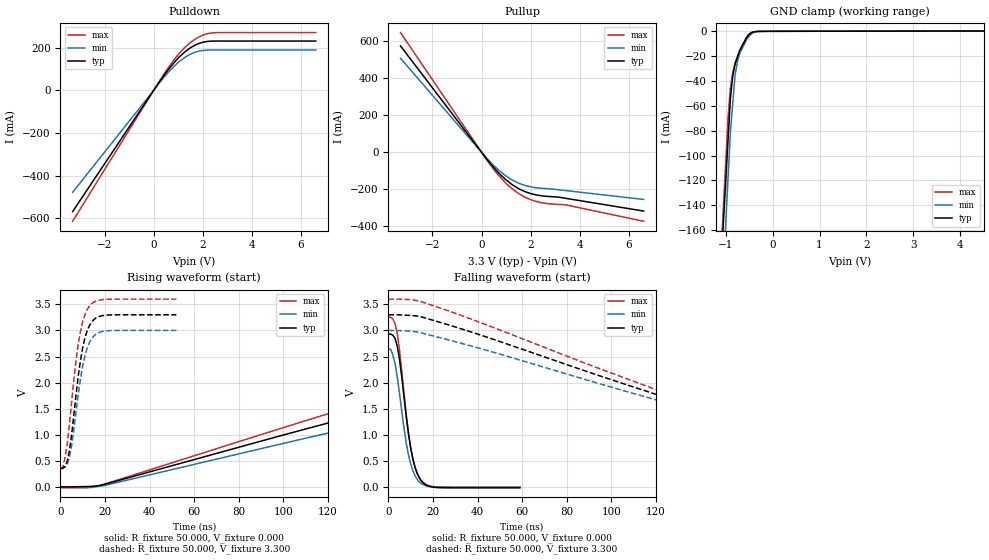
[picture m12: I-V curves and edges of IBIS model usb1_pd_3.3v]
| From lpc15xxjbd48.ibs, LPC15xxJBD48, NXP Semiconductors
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[Model]   usb1_pd_3.3v
Model_type I/O
Vinl=9.900E-01
Vinh=2.310E+00
Vref=0.000E+00
Rref=1.000E+06
Cref=0.000E+00
Vmeas=1.650E+00
C_comp   2.000E-12   2.000E-12   2.000E-12
[Voltage Range]   3.300E+00   3.000E+00   3.600E+00
[POWER Clamp Reference]   3.300E+00   3.000E+00   3.600E+00
[GND Clamp Reference]   0.000E+00   0.000E+00   0.000E+00
[Pullup Reference]   3.300E+00   3.000E+00   3.600E+00
[Pulldown Reference]   0.000E+00   0.000E+00   0.000E+00
[Temperature Range]   25   85   -40
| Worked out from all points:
|   slope of the pulldown table from 0 to 0.495 V, typ, clamps not added: 6.06 ohm
|   slope of the pullup table from 0 to 0.495 V, typ, clamps not added: 6.04 ohm
|   GND clamp passes 1 mA (typ) near -0.44 V on its own axis
|   rising waveform, R_fixture 50.000, V_fixture 0.000: 20-80 % time 164ns typ, 173ns min, 155ns max; typ from 0 V to 2.95 V
|   falling waveform, R_fixture 50.000, V_fixture 0.000: 20-80 % time 5.51ns typ, 5.54ns min, 5.45ns max; typ from 2.93 V to -0.014 V
|   rising waveform, R_fixture 50.000, V_fixture 3.300: 20-80 % time 5.37ns typ, 5.43ns min, 5.35ns max; typ from 0.352 V to 3.3 V
|   falling waveform, R_fixture 50.000, V_fixture 3.300: 20-80 % time 127ns typ, 132ns min, 123ns max; typ from 3.3 V to 0.352 V
[GND Clamp]
-3.3V     -1.665A    -1.867A    -1.78A
-950mV    -88mA      -118.7mA   -70.2mA
-900mV    -54.45mA   -81.5mA    -45.76mA
-850mV    -36.23mA   -58.43mA   -32.88mA
-800mV    -26.46mA   -35.35mA   -25.59mA
-750mV    -21mA      -24.36mA   -20.37mA
-700mV    -15.55mA   -17.9mA    -15.15mA
-550mV    -4.778mA   -6.346mA   -4.234mA
-450mV    -1.105mA   -1.932mA   -913.8uA
-350mV    -204.8uA   -365.7uA   -198.6uA
-150mV    -14.97uA   -25.94uA   -16.54uA
6.6V      390.1uA    400uA      390.5uA
[Power Clamp]
-3.3V     0A         0A         0A
0V        0A         0A         0A
3.3V      0A         0A         0A
6.6V      0A         0A         0A
[Pullup]
-3.3V     573.9mA    507.4mA    646.2mA
260mV     -45.14mA   -39.12mA   -50.35mA
720mV     -114.4mA   -98.69mA   -128mA
1.02V     -151.1mA   -130mA     -170.2mA
1.28V     -177.4mA   -151.7mA   -200.2mA
1.8V      -213.8mA   -180.2mA   -244.2mA
2.34V     -232.8mA   -193.1mA   -269.2mA
2.74V     -238.6mA   -196.9mA   -277.9mA
3.44V     -248.8mA   -206.9mA   -284.2mA
6.6V      -317.3mA   -254.6mA   -372.5mA
[Pulldown]
-3.3V     -569.7mA   -479mA     -615.1mA
420mV     69.92mA    61.22mA    76.39mA
1V        151.6mA    131.1mA    167.7mA
1.48V     198.8mA    169.2mA    223.1mA
1.94V     224mA      186.5mA    256.1mA
2.44V     231.7mA    189.6mA    270.6mA
6.6V      231.7mA    189.6mA    271.6mA
[Rising Waveform]
R_fixture = 50.000
V_fixture = 0.000
V_fixture_min = 0.000
V_fixture_max = 0.000
|  time   V(typ)   V(min)   V(max)
0s        30.69uV    94.86uV    -17.02mV
17ns      24.3mV     10.84mV    15.03mV
112ns     1.133V     953.6mV    1.296V
168ns     1.755V     1.487V     2.007V
223ns     2.307V     1.964V     2.631V
254ns     2.557V     2.193V     2.889V
293ns     2.745V     2.39V      3.061V
352ns     2.871V     2.537V     3.161V
417ns     2.923V     2.604V     3.203V
513ns     2.954V     2.642V     3.228V
[Falling Waveform]
R_fixture = 50.000
V_fixture = 0.000
V_fixture_min = 0.000
V_fixture_max = 0.000
|  time   V(typ)   V(min)   V(max)
0s        2.931V     2.642V     3.254V
2ns       2.91V      2.531V     3.22V
4ns       2.698V     2.112V     2.935V
5ns       2.449V     1.794V     2.626V
8ns       1.359V     851.9mV    1.398V
10ns      753.5mV    446mV      762.5mV
12ns      374.8mV    214.9mV    378.1mV
15ns      108.7mV    63.38mV    116mV
22ns      -8.347mV   2.621mV    5.036mV
59ns      -13.87mV   94.86uV    35.81uV
[Rising Waveform]
R_fixture = 50.000
V_fixture = 3.300
V_fixture_min = 3.000
V_fixture_max = 3.600
|  time   V(typ)   V(min)   V(max)
0s        351.9mV    365.5mV    361.3mV
1ns       353.9mV    365.5mV    360.4mV
2ns       389.9mV    379.4mV    553.4mV
4ns       689.2mV    561.4mV    1.191V
6ns       1.375V     1.095V     2.047V
8ns       2.128V     1.78V      2.74V
10ns      2.674V     2.324V     3.17V
13ns      3.093V     2.766V     3.467V
20ns      3.29V      2.988V     3.594V
52ns      3.3V       3V         3.6V
[Falling Waveform]
R_fixture = 50.000
V_fixture = 3.300
V_fixture_min = 3.000
V_fixture_max = 3.600
|  time   V(typ)   V(min)   V(max)
0s        3.3V       3V         3.6V
12ns      3.281V     2.977V     3.579V
24ns      3.145V     2.852V     3.419V
144ns     1.448V     1.388V     1.496V
184ns     925mV      936.1mV    906.2mV
206ns     672.8mV    712.6mV    636.6mV
225ns     529mV      571.6mV    504.3mV
249ns     437.8mV    471.3mV    427.9mV
285ns     381.7mV    403.2mV    384.3mV
339ns     351.9mV    365.5mV    361.3mV
[Ramp]
dV/dt_r   1.7668E+00/1.6350E-07   1.5807E+00/1.7195E-07   1.9467E+00/1.5631E-07
dV/dt_f   1.7689E+00/1.2734E-07   1.5807E+00/1.3210E-07   1.9432E+00/1.2325E-07
R_load = 50
